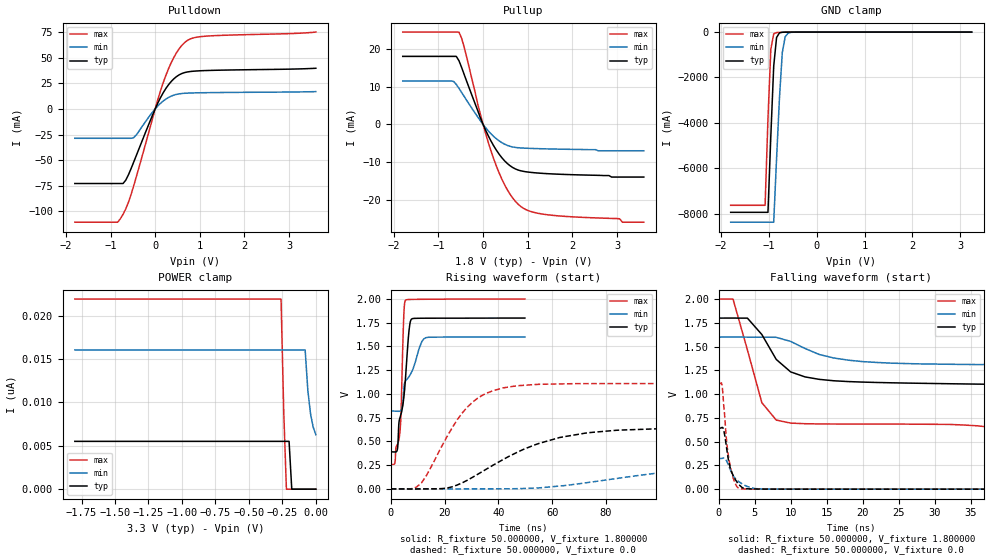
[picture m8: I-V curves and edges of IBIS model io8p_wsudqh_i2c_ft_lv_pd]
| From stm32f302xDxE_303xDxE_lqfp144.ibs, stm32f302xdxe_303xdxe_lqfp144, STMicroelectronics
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|   Model io8p_wsudqh_i2c_ft_lv_pd
[Model]  io8p_wsudqh_i2c_ft_lv_pd
Model_type I/O
Polarity   Non-Inverting
Enable   Active-Low
Vinl =   0.540000V
Vinh =   1.260000V
Vmeas =  0.900000V
Cref =   40.000000pF
Rref =   100.000000M
Vref =   0.0V
C_comp   0.0F   0.0F   0.0F
[Temperature Range]   25.000000   0.140000k   -40.000000
[Pullup Reference]   1.800000V   1.600000V   2.000000V
[Pulldown Reference]   0.0V   0.0V   0.0V
[POWER Clamp Reference]   3.300000V   2.700000V   3.600000V
[GND Clamp Reference]   0.0V   0.0V   0.0V
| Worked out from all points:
|   slope of the pulldown table from 0 to 0.27 V, typ, clamps not added: 12.4 ohm
|   slope of the pullup table from 0 to 0.27 V, typ, clamps not added: 42.7 ohm
|   GND clamp passes 1 mA (typ) near -0.61 V on its own axis
|   rising waveform, R_fixture 50.000000, V_fixture 1.800000: 20-80 % time 3.36ns typ, 5.5ns min, 1.18ns max; typ from 0.39 V to 1.8 V
|   rising waveform, R_fixture 50.000000, V_fixture 0.0: 20-80 % time 28.6ns typ, 60ns min, 14.6ns max; typ from 0 V to 0.642 V
|   falling waveform, R_fixture 50.000000, V_fixture 1.800000: 20-80 % time 95.2ns typ, 220ns min, 38.6ns max; typ from 1.8 V to 0.39 V
|   falling waveform, R_fixture 50.000000, V_fixture 0.0: 20-80 % time 1.17ns typ, 1.76ns min, 970ps max; typ from 0.642 V to 0 V
[Pulldown]
|Voltage   I(typ)   I(min)   I(max)
-1.8V     -72.82mA   -28.67mA   -110.6mA
-840mV    -72.82mA   -28.67mA   -110.6mA
-780mV    -72.82mA   -28.67mA   -107.2mA
-660mV    -69.63mA   -28.67mA   -97.65mA
-480mV    -51.79mA   -27.98mA   -74.89mA
0V        0A         0A         0A
240mV     19.98mA    9.621mA    32.82mA
420mV     29.47mA    13.52mA    50.45mA
660mV     35.49mA    15.27mA    64.82mA
840mV     36.76mA    15.6mA     69.15mA
1.14V     37.47mA    15.86mA    71.05mA
3.6V      39.71mA    16.9mA     75.01mA
[Pullup]
|Voltage   I(typ)   I(min)   I(max)
-1.8V     18.1mA     11.55mA    24.56mA
-720mV    18.1mA     11.55mA    24.56mA
-600mV    18.1mA     10.63mA    24.56mA
-540mV    16.94mA    9.592mA    24.54mA
-420mV    13.16mA    7.372mA    20.4mA
-60mV     1.723mA    986.2uA    2.671mA
240mV     -5.743mA   -3.225mA   -9.221mA
540mV     -10.36mA   -5.558mA   -17.32mA
840mV     -12.32mA   -6.245mA   -21.78mA
1.08V     -12.77mA   -6.379mA   -23.2mA
1.44V     -13.09mA   -6.504mA   -24.02mA
3.6V      -14mA      -7mA       -26mA
[GND_clamp]
|Voltage   I(typ)   I(min)   I(max)
-1.8V     -7.944A    -8.38A     -7.635A
-1.08V    -7.944A    -8.38A     -7.635A
-1.02V    -7.944A    -8.38A     -3.818A
-960mV    -4.573A    -8.38A     -759.3mA
-900mV    -1.502A    -8.38A     -75.05mA
-840mV    -238mA     -5.574A    -20.41mA
-780mV    -36.14mA   -2.918A    -12.66mA
-720mV    -8.013mA   -894.2mA   -8.079mA
-660mV    -2.394mA   -209.5mA   -4.371mA
-600mV    -735.9uA   -49.63mA   -1.768mA
-420mV    -17.12uA   -720.6uA   -21.31uA
3.24V     77.98uA    62.12uA    84.87uA
[POWER_clamp]
|Voltage   I(typ)   I(min)   I(max)
-1.8V     5.515nA    16.06nA    21.93nA
-260mV    5.515nA    16.06nA    21.93nA
-240mV    5.515nA    16.06nA    8.985nA
-220mV    5.515nA    16.06nA    0A
-200mV    5.515nA    16.06nA    0A
-180mV    0A         16.06nA    0A
-80mV     0A         16.06nA    0A
-60mV     0A         11.42nA    0A
-40mV     0A         8.703nA    0A
-20mV     0A         7.161nA    0A
0V        0A         6.282nA    0A
[Ramp]
| variable   typ   min   max
dV/dt_r  0.38519/28.57415n   0.19271/59.37804n   0.66540/14.53052n
dV/dt_f  0.84282/94.85174n   0.39610/0.18875u   1.04475/38.27004n
R_load = 50.000000
[Rising Waveform]
R_fixture= 50.000000
V_fixture= 1.800000
V_fixture_min= 1.600000
V_fixture_max= 2.000000
|time   V(typ)   V(min)   V(max)
0s        389.8mV    820.1mV    257.9mV
1.502ns   388.7mV    818.9mV    267.3mV
2.402ns   406mV      817.4mV    463.1mV
3.504ns   754.6mV    819.7mV    617.1mV
4.805ns   944mV      1.021V     1.781V
5.506ns   1.169V     1.137V     1.986V
6.807ns   1.666V     1.182V     1.995V
8.008ns   1.792V     1.246V     1.996V
13.11ns   1.798V     1.592V     1.997V
49.85ns   1.799V     1.599V     1.999V
[Rising Waveform]
R_fixture= 50.000000
V_fixture= 0.0
V_fixture_min= 0.0
V_fixture_max= 0.0
|time   V(typ)   V(min)   V(max)
0s        944.5pV    19.89nV    679.9pV
11.41ns   -341.1uV   -775.8uV   62.07mV
24.72ns   40.75mV    -73.89uV   728.6mV
32.33ns   153.8mV    6.348uV    955.5mV
41.84ns   310.5mV    426.2uV    1.064V
55.16ns   479.2mV    10.39mV    1.101V
85.59ns   619.5mV    115.9mV    1.109V
131.2ns   641.8mV    255.7mV    1.109V
182.6ns   642mV      309mV      1.109V
947.1ns   642mV      322.4mV    1.109V
[Falling Waveform]
R_fixture= 50.000000
V_fixture= 1.800000
V_fixture_min= 1.600000
V_fixture_max= 2.000000
|time   V(typ)   V(min)   V(max)
0s        1.799V     1.599V     1.999V
2.002ns   1.799V     1.601V     1.999V
6.006ns   1.626V     1.599V     909.6mV
8.008ns   1.364V     1.597V     726.5mV
22.02ns   1.122V     1.332V     684.8mV
80.08ns   943mV      1.301V     292.8mV
114.1ns   555.5mV    1.295V     267.3mV
166.2ns   422.1mV    1.204V     259.5mV
338.3ns   390.5mV    850.7mV    257.9mV
997ns     389.8mV    820.1mV    257.9mV
[Falling Waveform]
R_fixture= 50.000000
V_fixture= 0.0
V_fixture_min= 0.0
V_fixture_max= 0.0
|time   V(typ)   V(min)   V(max)
0s        642mV      322.4mV    1.109V
500.5ps   650mV      323.7mV    1.085V
700.7ps   623.4mV    327.3mV    888.6mV
1.101ns   438.1mV    298.5mV    512mV
1.502ns   257.3mV    226.6mV    284.3mV
2.202ns   117.2mV    122.3mV    75.15mV
2.803ns   49.33mV    79.11mV    8.524mV
3.704ns   6.507mV    37.95mV    1.895mV
5.906ns   1.042mV    1.776mV    570.1uV
49.85ns   944.5pV    19.89nV    679.9pV
